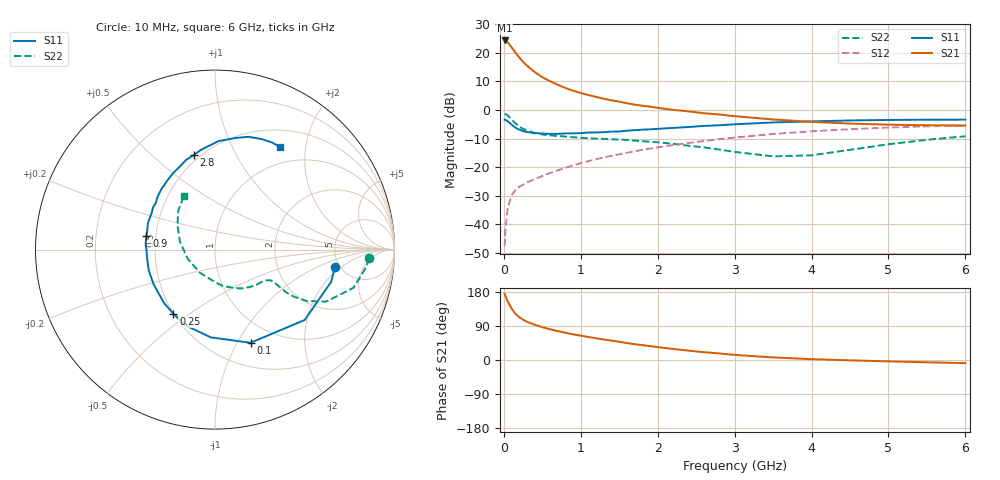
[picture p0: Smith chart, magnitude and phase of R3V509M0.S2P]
! SIEMENS Small Signal Semiconductors
! BFR181
! Si NPN RF Bipolar Junction Transistor in SOT23
! VCE = 0.5 V  IC = 9 mA
! Common Emitter S-Parameters:  May  1996
# GHz  S  MA  R  50
!  f  S11  S21  S12  S22
! GHz  MAG  ANG  MAG  ANG  MAG  ANG  MAG  ANG
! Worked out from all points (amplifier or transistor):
!   36 points, 10 MHz to 6 GHz, reference 50 ohm
!   highest |S21| = 24.4 dB at 10 MHz (marker M1)
!   |S21| within 3 dB of that: start of sweep to 117.3 MHz
!   unconditionally stable (mu >= 1): start of sweep to 11.13 MHz; 263.1 MHz to end of sweep
!   at 250 MHz: K = 0.97, MSG = 21.6 dB, |S12| = -26.2 dB
!   at 1.4 GHz: K = 1.60, MAG = 5.2 dB, |S12| = -16.1 dB
!   at 6 GHz: K = 1.21, MAG = -2.8 dB, |S12| = -5.4 dB
!   S11 on the Smith chart (normalised r, x): 10 MHz: 4.57, -1.62; 100 MHz: 0.76, -1.14; 250 MHz: 0.50, -0.43; 900 MHz: 0.44, +0.08; 2.8 GHz: 0.46, +0.69; 6 GHz: 0.73, +1.55
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0.01  0.6758 -8.2  16.54 174.8  0.0041 83.8  0.8593 -3.2
0.02  0.6716 -15.5  16.32 169.4  0.0078 81.7  0.848 -6.6
0.05  0.6352 -38.1  15.35 154.9  0.0188 71.4  0.8005 -15.4
0.1  0.5557 -69.1  12.62 136.0  0.0318 60.5  0.6837 -25.1
0.15  0.4894 -92.8  10.16 122.1  0.0393 54.5  0.585 -29.3
0.2  0.4533 -110.8  8.343 113.0  0.0449 52.0  0.5137 -30.8
0.25  0.4261 -123.0  6.991 106.2  0.0489 51.5  0.4667 -31.0
0.3  0.4107 -134.0  5.999 101.0  0.0537 52.0  0.438 -30.5
0.4  0.3928 -150.8  4.629 93.0  0.0613 53.5  0.3956 -29.5
0.5  0.3871 -162.2  3.752 86.5  0.0697 55.4  0.3712 -28.9
0.6  0.3818 -170.9  3.196 81.3  0.0784 57.3  0.359 -28.9
0.7  0.3813 -178.9  2.772 76.3  0.0875 58.8  0.3497 -29.2
0.9  0.3891 169.0  2.176 67.8  0.107 60.1  0.3332 -31.0
1.1  0.4019 158.5  1.825 60.7  0.1271 60.7  0.3203 -33.9
1.3  0.4081 149.6  1.575 54.1  0.1473 60.3  0.3113 -36.9
1.7  0.4426 134.1  1.241 41.6  0.1879 58.5  0.2903 -44.5
2.2  0.4855 118.8  1.003 29.2  0.2427 54.2  0.2554 -57.9
2.8  0.5399 102.7  0.833 17.3  0.308 47.7  0.2026 -79.7
3.5  0.6045 88.2  0.682 6.8  0.3794 38.6  0.1539 -122.8
4.5  0.6554 73.5  0.577 -0.9  0.4601 24.4  0.2003 167.3
5.5  0.6757 62.3  0.54 -6.0  0.516 11.3  0.3003 132.7
6  0.6774 57.9  0.533 -8.3  0.5358 4.7  0.3457 120.1
